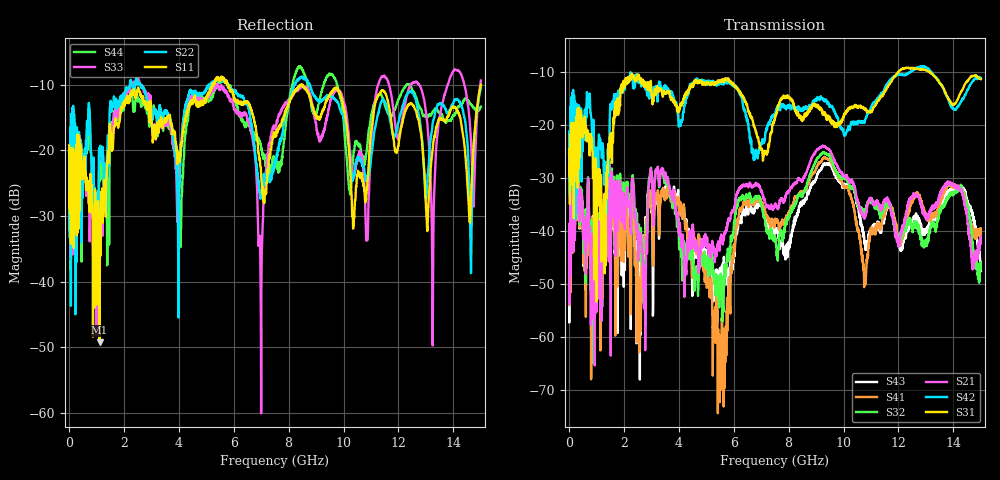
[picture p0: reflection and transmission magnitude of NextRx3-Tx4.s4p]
!  = SDD11
!  = SDD12
!  = SDC11
!  = SDC12
!  = SDD21
!  = SDD22
!  = SDC21
!  = SDC22
!  = SCD11
!  = SCD12
!  = SCC11
!  = SCC12
!  = SCD21
!  = SCD22
!  = SCC21
!  = SCC22
! FILE: N:\QM 2007\Prüfprotokolle\Highspeed\Konfektionierte Ltg\L45593-D106\D30\8216\0002\Next  Platine 1\NextRx3-Tx4.s4p
# MHz S DB R 50.00
! FREQ  S11  S12  S13  S14
!  S21  S22  S23  S24
!  S31  S32  S33  S34
!  S41  S42  S43  S44
!  DB  ANG  DB  ANG  DB  ANG  DB  ANG
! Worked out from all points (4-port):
!   2999 points, 10 MHz to 15 GHz, reference 50 ohm
!   strongest paths, dB at 10 MHz, 3.755 GHz, 7.505 GHz, 11.26 GHz, 15 GHz:
!     S31: -24.5, -15.2, -18.7, -15.4, -11.3
!     S42: -25.2, -13.7, -18.2, -14.9, -11.2
!     S21: -44.2, -33.8, -34.9, -34.7, -41.0
!     S32: -42.7, -34.5, -40.9, -35.4, -47.0
!     S41: -47.6, -34.5, -38.1, -38.9, -40.5
!     S43: -52.4, -32.9, -40.2, -38.4, -47.5
!   lowest |S11| = -49.2 dB at 1.12 GHz (marker M1), VSWR 1.01, Z = 49.7 - j0.0474 ohm
!   |S11| at or under -10 dB: start of sweep to 5.214 GHz; 5.776 GHz to 8.447 GHz (2.671 GHz wide, 37.6 % of centre); 8.49 GHz to end of sweep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
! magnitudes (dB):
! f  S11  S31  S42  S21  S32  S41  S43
! 10 MHz  -19.2  -24.5  -25.2  -44.2  -42.7  -47.6  -52.4
! 1.12 GHz  -49.2  -28.3  -23.6  -45.2  -46.1  -42.7  -44.7
! 3.865 GHz  -17.4  -16.2  -15.6  -35.5  -36.7  -34.5  -33.5
! 5.49 GHz  -9.4  -11.6  -12.2  -43.7  -49.7  -61.6  -47.4
! 6.965 GHz  -22.1  -24.1  -23.6  -31.8  -34.0  -33.8  -34.3
! 9.335 GHz  -12.8  -17.9  -15.4  -24.0  -25.3  -26.2  -27.4
! 15 GHz  -10.0  -11.3  -11.2  -41.0  -47.0  -40.5  -47.5
